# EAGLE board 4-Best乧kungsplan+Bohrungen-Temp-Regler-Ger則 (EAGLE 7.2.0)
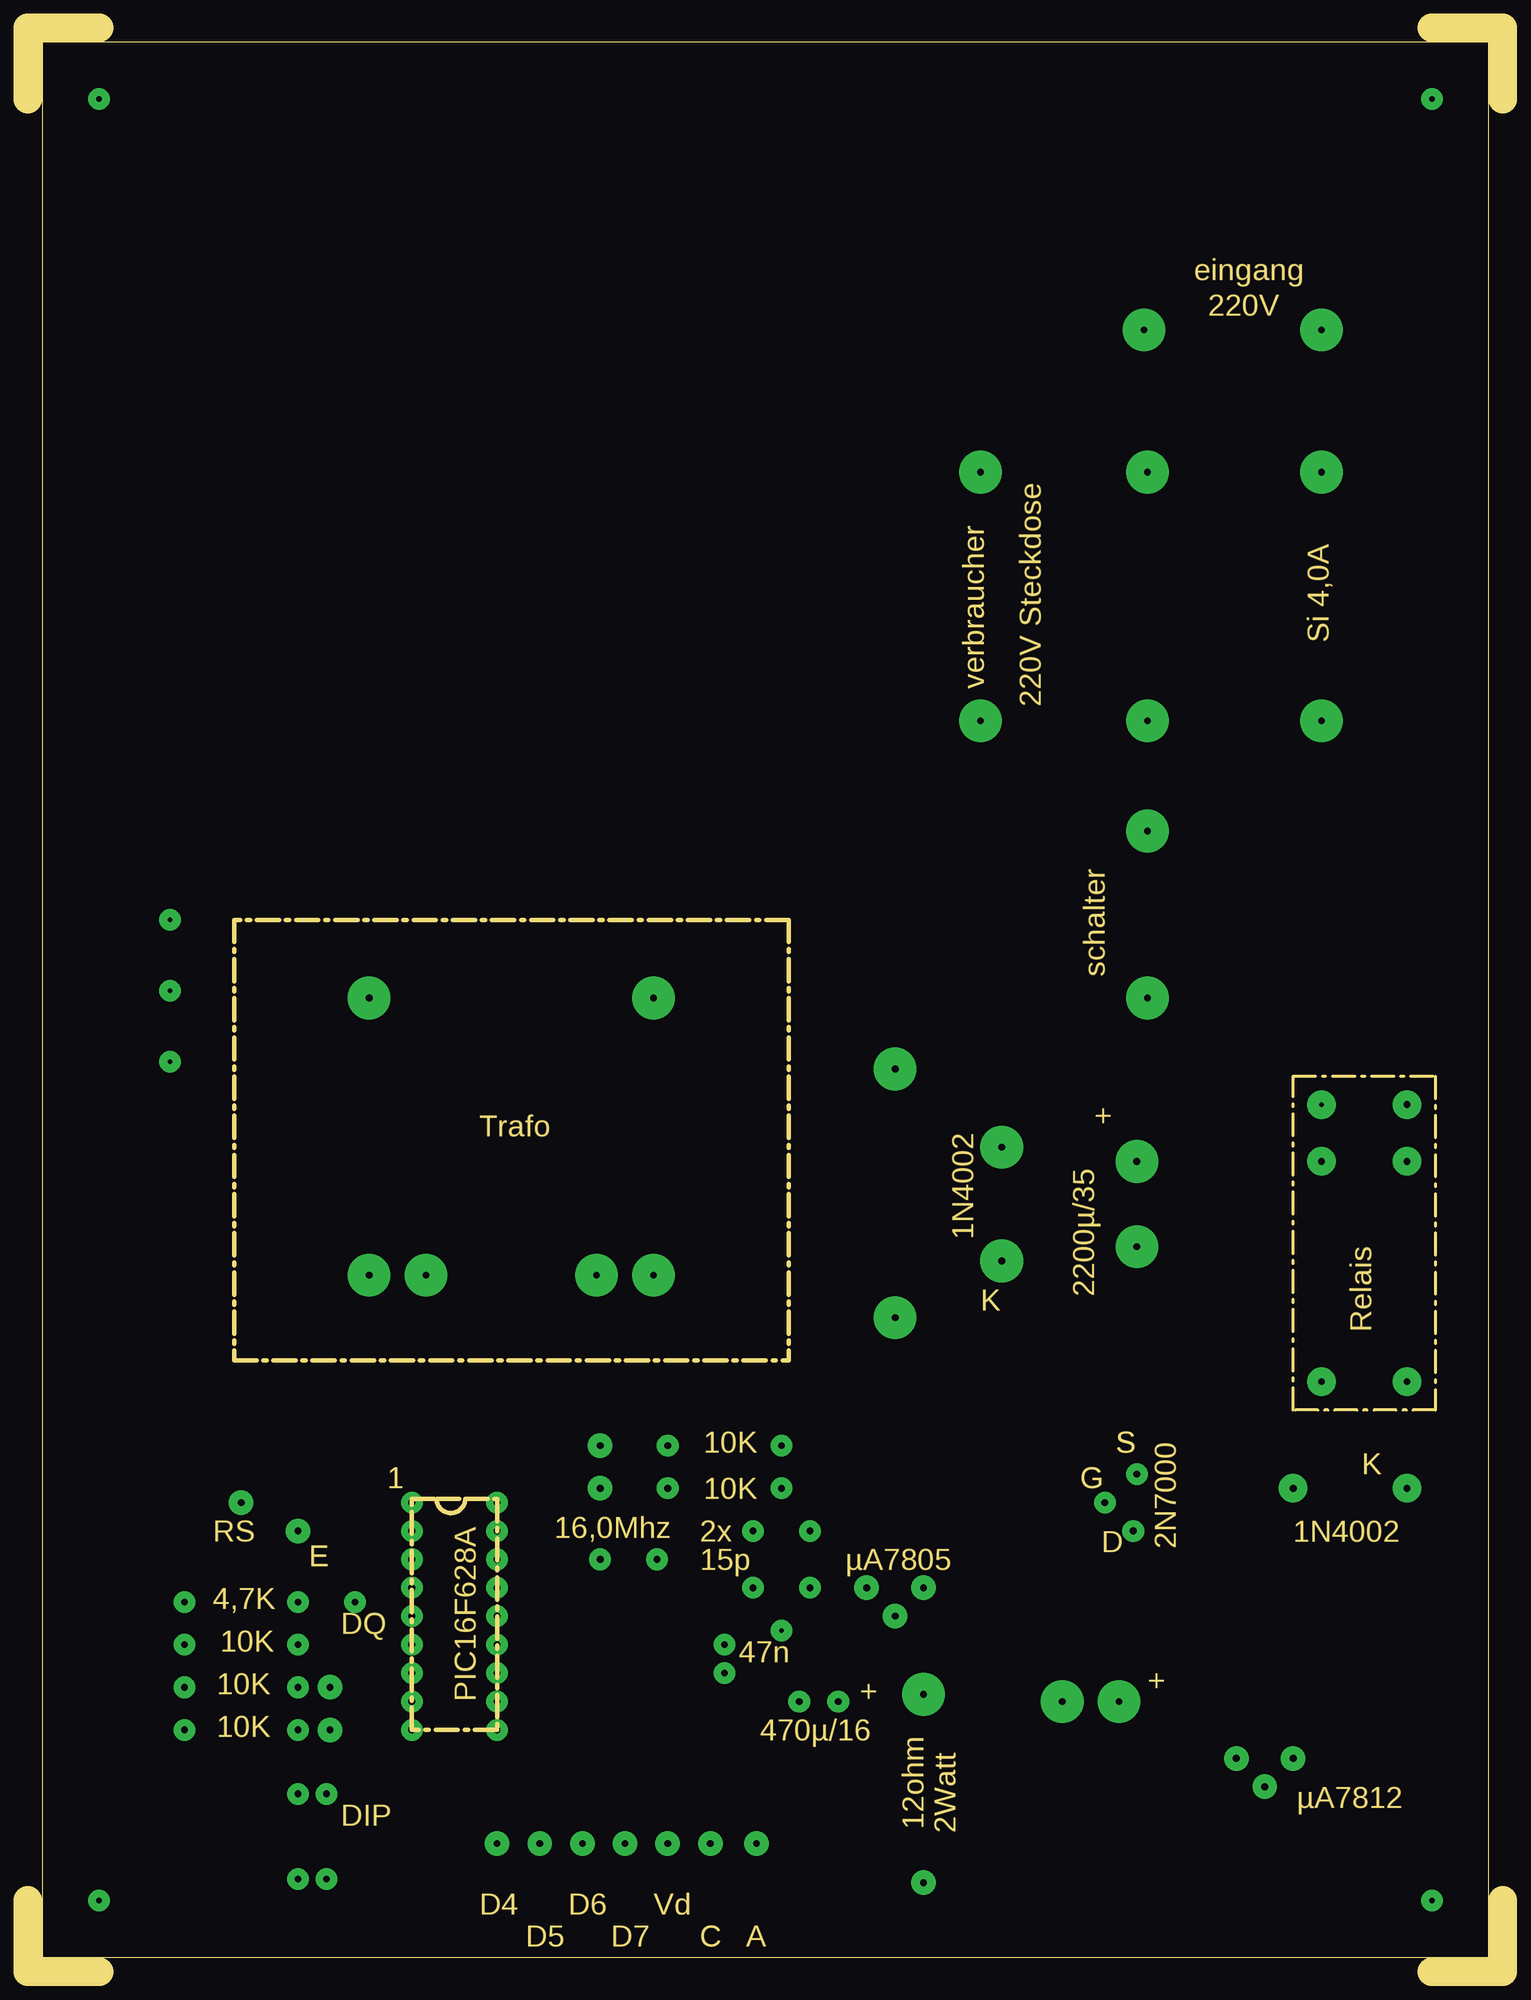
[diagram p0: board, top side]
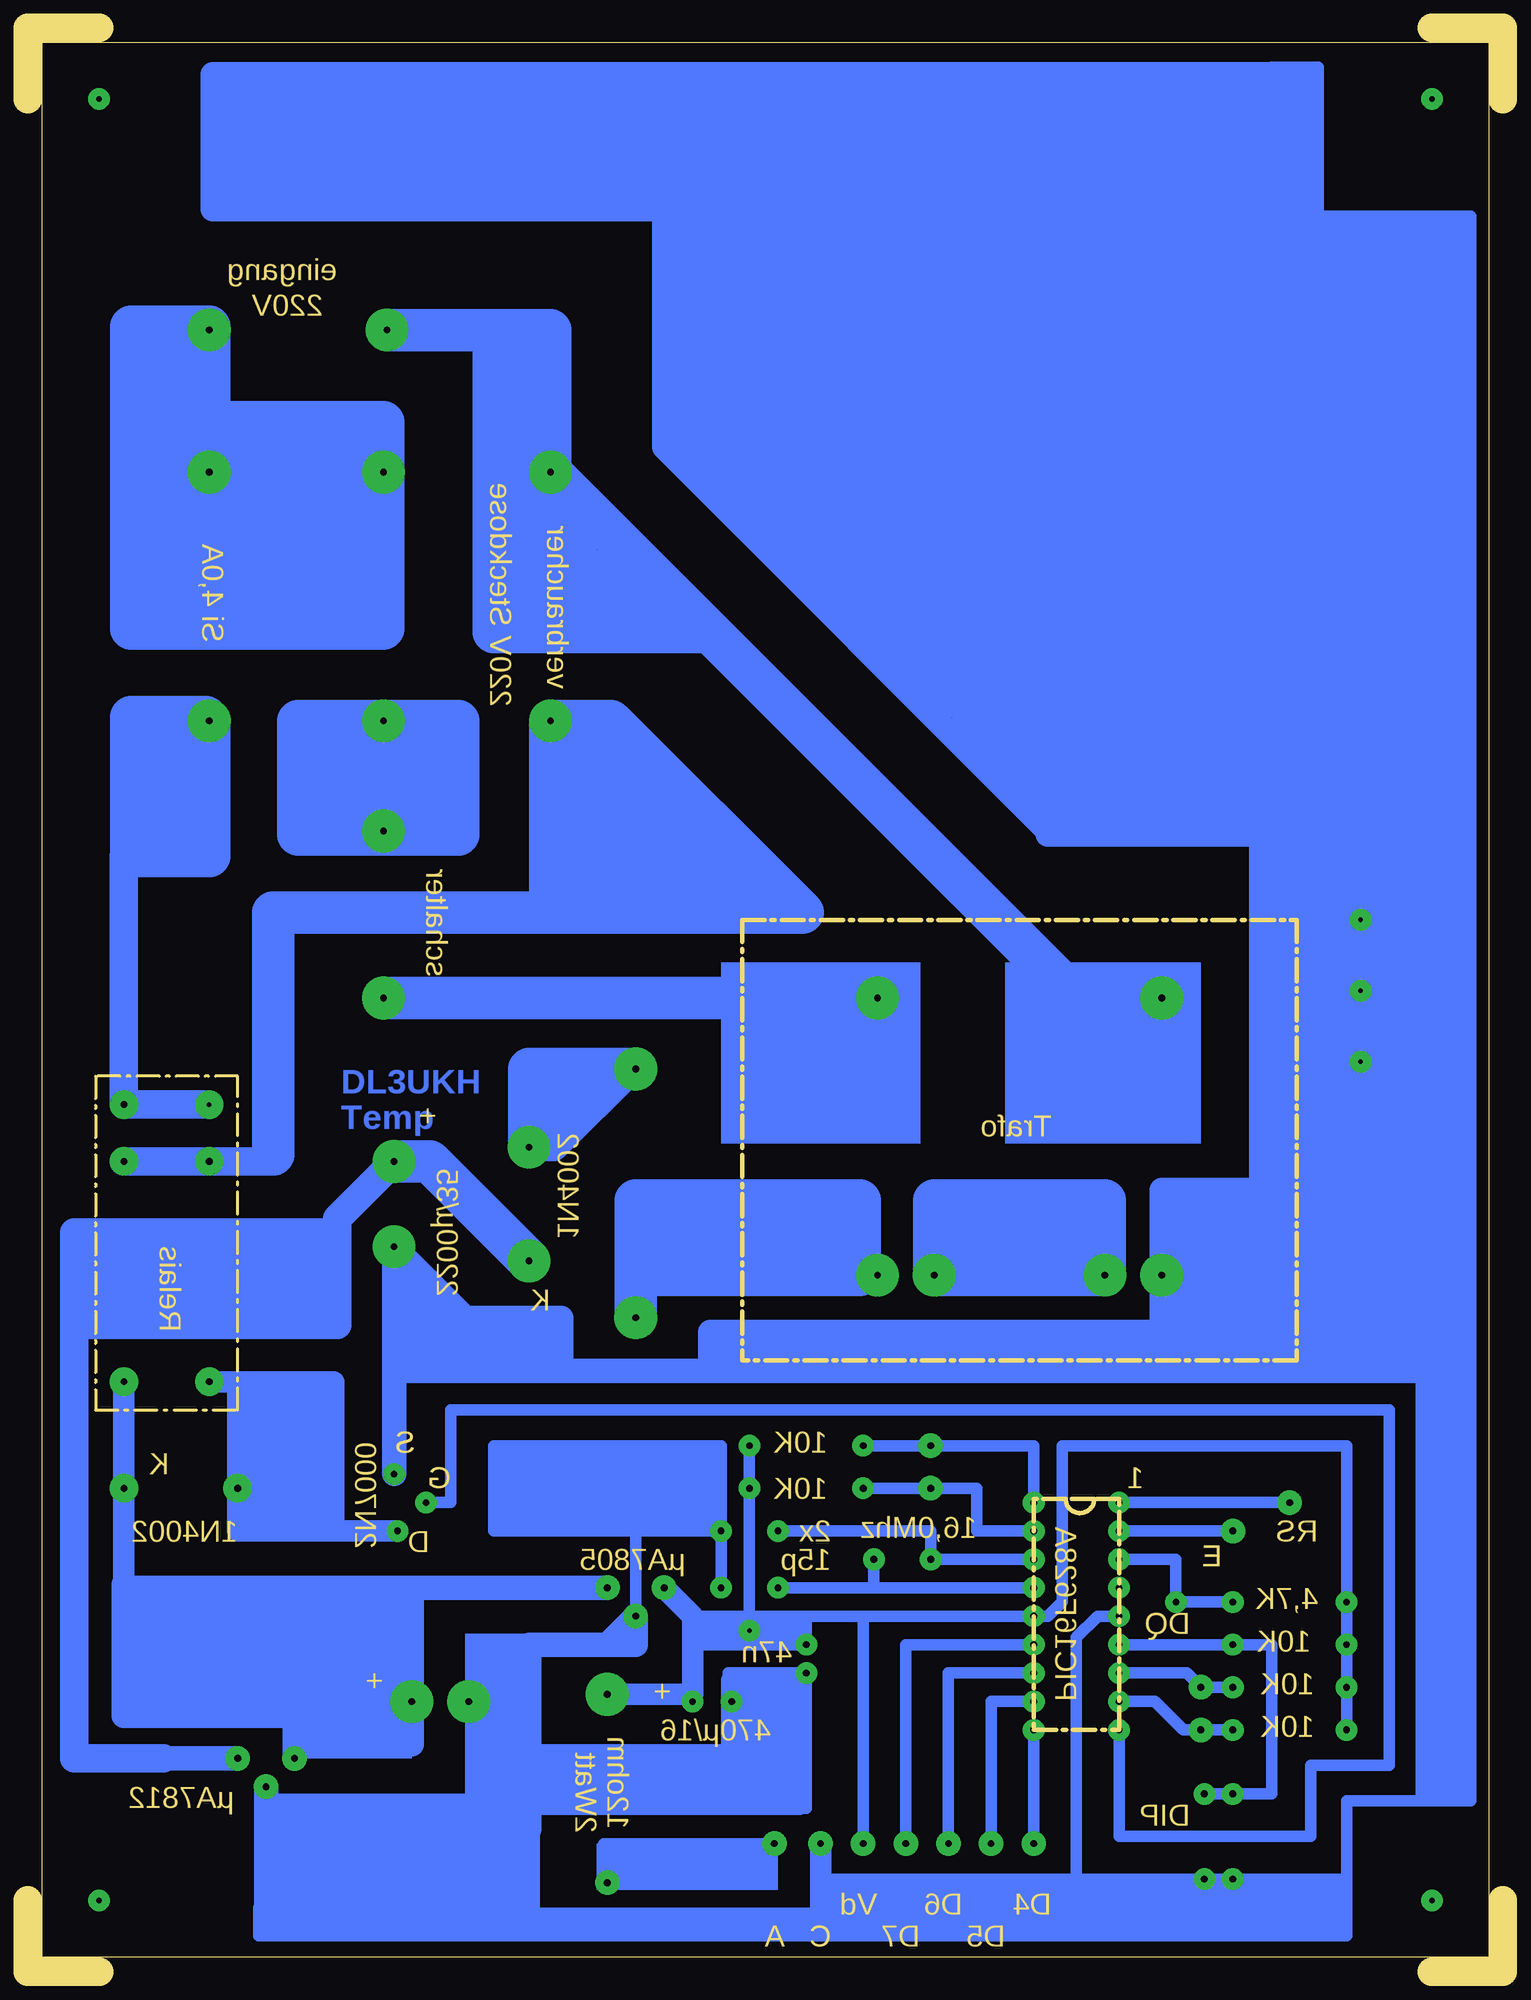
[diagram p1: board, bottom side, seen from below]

Size 131.76 x 173.67 mm. Coordinates in mm from the lower left corner, seen from the top.
Outline: 0,6.35 0,0 6.35,0
Outline: 131.76,6.35 131.76,0 125.41,0
Outline: 0,167.32 0,173.67 6.35,173.67
Outline: 131.76,167.32 131.76,173.67 125.41,173.67
Outline: 36.51,42.23 34.29,42.23 34.29,21.59 41.91,21.59 41.91,42.23 39.05,42.23
Outline: 36.51,42.23 39.05,42.23
Outline: 36.51,42.23 arc180 39.05,42.23
Outline: 1.27,1.27 130.49,1.27 130.49,172.4 1.27,172.4 1.27,1.27
Outline: 67.94,93.98 67.94,54.61 18.41,54.61 18.41,93.98 67.94,93.98
Outline: 113.03,80.01 125.73,80.01 125.73,50.17 113.03,50.17 113.03,80.01
Copper layers (1*16): Top 0.035mm / dielectric 1.5mm / Bottom 0.035mm
Design rules "default": minimum track width 10mil, minimum drill 24mil, track to track 8mil, track to pad 8mil, pad to pad 8mil, via to via 8mil, smd to smd 8mil, copper to edge 40mil, drill to drill 8mil, minimum pad ring 10mil, minimum via ring 8mil, stop-mask expansion 4mil, vias tented up to drill 0mil, thermal gap 10mil

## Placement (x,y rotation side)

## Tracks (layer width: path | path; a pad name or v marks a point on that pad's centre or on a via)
S$1  (via drill 0.5 pad 1.93)
  other vias: 6.35,6.35
S$2  (via drill 0.5 pad 1.93)
  other vias: 6.35,167.32
S$3  (via drill 0.5 pad 1.93)
  other vias: 125.41,167.32
S$4  (via drill 0.5 pad 1.93)
  other vias: 125.41,6.35
S$5  (via drill 0.6 pad 1.93)
  other vias: 72.39,24.13
S$6  (via drill 0.6 pad 3.81)
  Bottom 3.81: v35.56,62.23 v50.8,62.23 50.8,68.9 35.56,68.9 v35.56,62.23
S$7  (via drill 0.6 pad 3.81)
  Bottom 3.81: v100.01,111.76 v100.01,101.92 | v100.01,111.76 100.33,111.76 107.63,111.76 107.63,101.6 93.34,101.6 93.34,111.76 v100.01,111.76
S$8  (via drill 0.6 pad 3.81)
  Bottom 3.81: 77.47,61.91 77.47,62.23 57.47,62.23 57.47,68.9 77.47,68.9 77.47,61.91 | 77.47,61.91 v77.47,58.42
S$9  (via drill 0.6 pad 1.93, 0.6 pad 2.18)
  Bottom 1.016: v41.91,41.91 41.91,46.99 v51.12,46.99 v57.15,46.99
S$10  (via drill 0.6 pad 3.81)
  other vias: 100.01,86.99
S$11  (via drill 0.6 pad 3.81)
  Bottom 3.81: v55.88,86.99 100.01,86.99
S$12  (via drill 0.4 pad 2.54, 0.6 pad 2.54)
  Bottom 2.54: v115.57,77.47 v123.19,77.47 123.19,99.69
S$13  (via drill 0.6 pad 3.81)
  Bottom 3.81: v115.57,111.76 115.57,99.69 122.55,99.69
S$14  (via drill 0.6 pad 2.18)
  Bottom 1.016: v65.09,11.43 80.33,11.43 v80.01,7.94
S$15
  Bottom 3.81: 90.17,146.37 90.17,119.7 71.44,119.7
S$16  (via drill 0.6 pad 1.93)
  Bottom 1.016: v34.29,41.91 19.05,41.91
S$17  (via drill 0.6 pad 1.93, 0.6 pad 2.18)
  Bottom 1.016: v34.29,39.37 v24.13,39.37
S$18  (via drill 0.6 pad 3.81)
  Bottom 3.81: v99.69,146.69 85.09,146.69 v85.09,133.99 38.1,86.99 v30.48,86.99
S$19  (via drill 0.6 pad 3.81)
  other vias: 55.88,62.23
S$20  (via drill 0.6 pad 1.93)
  other vias: 34.29,34.29
S$21  (via drill 0.6 pad 1.93)
  Bottom 1.016: v34.29,31.75 36.2,31.75 38.1,29.84 38.1,12.38
S$22  (via drill 0.6 pad 1.93)
  Bottom 1.016: v34.29,21.59 34.29,12.06 17.14,12.06 17.14,18.41 10.16,18.41 10.16,50.17 93.98,50.17 93.98,41.91 v96.2,41.91
S$23  (via drill 0.6 pad 1.93, 0.6 pad 2.18)
  Bottom 1.016: v24.13,25.4 v26.99,25.4 28.26,26.67 v34.29,26.67
S$24
  Bottom 2.184: 30.8,57.15 70.8,57.15 70.8,54.29
S$25  (via drill 0.6 pad 1.93)
  other vias: 67.31,43.18
S$26  (via drill 0.6 pad 1.93, 0.6 pad 2.18)
  Bottom 1.016: 60.96,5.71 60.96,5.4 | v26.67,8.26 60.96,8.26
  Bottom 1.93: v60.96,11.43 60.96,8.26 60.96,5.71
S$27  (via drill 0.6 pad 1.93, 0.6 pad 2.18)
  Bottom 1.016: v41.91,39.37 46.99,39.37 46.99,43.18 v51.12,43.18 v57.15,43.18
S$28  (via drill 0.6 pad 1.93)
  Bottom 1.016: v41.91,36.83 v51.12,36.83 51.12,39.37 v64.77,39.37
S$29  (via drill 0.6 pad 1.93)
  Bottom 1.016: v41.91,34.29 56.2,34.29 | 56.2,34.29 v56.2,36.83 | 56.2,34.29 v64.77,34.29
S$30  (via drill 0.6 pad 1.93)
  Bottom 1.016: v34.29,29.21 v24.13,29.21 20.64,29.21 20.64,15.88 v26.67,15.88
S$31  (via drill 0.6 pad 1.93, 0.6 pad 2.18)
  Bottom 1.016: v41.91,29.21 53.34,29.21 v53.34,11.43
S$32  (via drill 0.6 pad 1.93, 0.6 pad 2.18)
  Bottom 1.016: v41.91,26.67 49.53,26.67 v49.53,11.43
S$33  (via drill 0.6 pad 1.93, 0.6 pad 2.18)
  Bottom 1.016: v41.91,24.13 45.72,24.13 v45.72,11.43
S$34  (via drill 0.6 pad 1.93, 0.6 pad 2.18)
  Bottom 1.016: v41.91,21.59 v41.91,11.43
S$35  (via drill 0.6 pad 1.93, 0.6 pad 2.18)
  Bottom 1.016: v24.13,21.59 v26.99,21.59 28.57,21.59 31.11,24.13 v34.29,24.13
S$36  (via drill 0.6 pad 3.81)
  Bottom 2.54: 77.79,80.64 84.77,73.66 87.31,73.66
  Bottom 3.81: v77.47,80.64 77.79,80.64 86.99,80.64 v86.99,73.66
S$37  (via drill 0.6 pad 1.93)
  other vias: 24.13,15.88
S$38  (via drill 0.6 pad 3.81)
  Bottom 2.184: v92.39,24.13 87.31,24.13
S$39  (via drill 0.6 pad 3.81)
  Bottom 3.81: 85.09,94.61 109.85,94.61 109.85,73.02 | 85.09,94.61 v85.09,111.76 79.69,111.76 62.55,94.61 85.09,94.61
S$40  (via drill 0.6 pad 2.18, 0.6 pad 3.81)
  Bottom 2.184: v113.03,19.05 119.7,19.05
  Bottom 2.54: 127.63,60.96 104.14,60.96 | 127.63,57.79 127.63,19.05 119.7,19.05 | 127.63,57.79 127.63,59.37 127.63,60.96 | 104.14,60.96 104.14,66.04 | 104.14,66.04 104.14,67.31 v99.06,72.39 | 104.14,60.96 104.14,57.79 127.63,57.79 | 104.14,66.04 127.63,66.04 127.63,60.96
  Bottom 3.81: v99.06,72.39 95.88,72.39 v86.99,63.5
S$41  (via drill 0.6 pad 1.93, 0.6 pad 2.18)
  Bottom 1.016: 21.59,53.34 7.3,53.34 | 7.3,53.34 7.3,15.24 | 7.3,15.24 13.97,15.24 13.97,8.26 | 62.23,24.13 v62.23,26.67 69.21,26.67 69.21,24.13 | 62.23,24.13 v68.9,24.13 | v69.85,39.37 v69.85,34.29 | 77.47,39.37 v69.85,39.37 | v77.47,31.75 77.47,39.37 | 86.99,5.08 86.99,13.02 | 38.1,5.08 86.99,5.08 | 38.1,5.08 38.1,12.06 | 86.99,5.08 111.12,5.08 | 62.23,24.13 62.23,14.61 69.21,14.61 | 26.67,5.08 24.13,5.08 | 24.13,5.08 13.97,5.08 | v24.13,8.26 26.67,8.26 26.67,5.08 | 38.1,5.08 26.67,5.08 | 13.97,8.26 13.97,5.08 | v24.13,8.26 24.13,5.08 | v69.85,39.37 69.85,46.99 90.17,46.99 90.17,39.37 77.47,39.37 | v24.13,8.26 13.97,8.26 | 7.3,15.24 2.86,15.24 2.86,53.34 | 2.86,53.34 7.3,53.34 | 2.86,53.34 2.86,156.84 16.51,156.84 16.51,170.18 20.64,170.18 | 13.97,5.08 13.97,3.17 111.12,3.17 111.12,5.71
  Bottom 1.93: 68.9,19.37 v68.9,24.13 68.9,26.04 | 68.9,19.37 86.68,19.37 | 68.9,19.37 68.9,14.92 | 86.99,29.21 86.99,24.13 | 68.9,14.92 86.99,14.92 | 68.9,14.92 62.87,14.92
  Bottom 2.184: 110.49,12.7 v110.49,16.51 | 80.01,29.21 v77.47,31.75 77.47,29.21 80.01,29.21 | 80.01,29.21 86.99,29.21 86.99,14.92 86.99,13.02 86.99,12.7 110.49,12.7 | 110.49,12.7 110.49,5.71
S$42  (via drill 0.6 pad 2.18, 0.6 pad 2.54, 0.6 pad 3.81)
  Bottom 1.016: v80.01,34.29 82.55,34.29
  Bottom 1.93: v123.19,52.71 123.19,34.61 123.19,29.21 115.57,29.21
  Bottom 2.184: 115.57,22.86 115.57,29.21 | v97.47,24.13 97.47,34.29 | 107.95,22.86 v107.95,19.05 | 107.95,22.86 115.57,22.86 | 107.95,22.86 97.47,22.86 v97.47,24.13 | v97.47,24.13 97.47,20.32 | 97.47,34.29 v80.01,34.29 | 97.47,34.29 123.19,34.29 | 123.19,34.29 123.19,34.61 | 115.57,22.86 123.19,22.86 123.19,34.29
S$43  (via drill 0.6 pad 1.93, 0.6 pad 2.54)
  Bottom 1.93: 104.46,39.37 104.46,52.71 113.03,52.71 | 104.46,39.37 103.82,39.37 v98.74,39.37 | 113.03,52.71 v115.57,52.71 | 113.03,52.71 v113.03,43.18 113.03,39.37 104.46,39.37
S$44  (via drill 0.6 pad 2.54)
  Bottom 2.54: v123.19,72.39 v115.57,72.39 109.85,72.39
S$45
  Bottom 3.81: 115.89,112.08 122.55,112.08 122.55,100.01
S$46  (via drill 0.6 pad 1.93, 0.6 pad 2.18)
  Bottom 1.016: v13.97,21.59 v13.97,33.02 13.97,46.99 39.37,46.99 39.37,33.02 40.64,31.75 v41.91,31.75 57.15,31.75 | 57.15,31.75 62.23,31.75 | 62.23,31.75 67.31,31.75 | 67.31,31.75 72.07,31.75 | 62.23,31.75 v62.23,29.21 72.07,29.21 | 57.15,31.75 v57.15,11.43 | v67.31,46.99 67.31,31.75
S$47  (via drill 0.6 pad 2.54)
  other vias: 123.19,43.18
S$48  (via drill 0.6 pad 3.81)
  Bottom 3.81: 115.57,147 122.55,147 122.55,133.99 | v115.57,146.69 v115.57,133.99 | v115.57,133.99 v100.01,133.99 | v115.57,133.99 122.55,133.99 | 122.55,133.99 122.55,120.02 100.01,120.02 100.01,138.43 114.3,138.43
S$49  (via drill 0.4 pad 1.93)
  other vias: 12.7,93.98
S$50  (via drill 0.4 pad 1.93)
  other vias: 12.7,87.63
S$51  (via drill 0.4 pad 1.93)
  other vias: 12.7,81.28
S$52  (via drill 0.6 pad 2.18, 0.6 pad 3.81)
  Bottom 1.93: v74.93,34.29 72.39,31.75 72.39,24.77 v80.01,24.77
S$53  (via drill 0.4 pad 1.93)
  other vias: 67.31,30.48
S$56  (via drill 0.6 pad 2.18)
  other vias: 19.05,41.91
S$58  (via drill 0.6 pad 1.93)
  other vias: 13.97,29.21
S$59  (via drill 0.6 pad 1.93, 0.6 pad 3.81)
  Bottom 1.016: v30.48,62.23 30.48,62.55
  Bottom 2.184: 99.06,53.66 v99.06,64.77 92.71,58.42 84.14,58.42 84.14,53.66 | 30.48,53.98 v30.48,62.23 | 30.48,53.66 84.14,53.66 | 84.14,53.66 99.06,53.66 | 99.06,53.66 v99.06,44.45 | v30.48,62.23 21.59,62.23 | 21.59,69.85 21.59,62.23 | v30.48,62.23 30.48,69.85 21.59,69.85 | 21.59,62.23 21.59,53.98 30.48,53.98 | 30.48,53.66 30.48,53.98 | 7.94,53.66 30.48,53.66 | 21.59,69.85 21.59,101.6 | 3.81,120.02 21.59,120.02 21.59,101.6 | 21.59,101.6 40.64,101.6 40.64,101.92 74.93,136.21 74.93,157.48 115.25,157.48 115.25,169.55 19.05,169.55
S$60  (via drill 0.6 pad 1.93)
  other vias: 13.97,25.4
S$63  (via drill 0.6 pad 1.93)
  Bottom 1.016: v24.13,33.02 v29.21,33.02 29.21,36.83 v34.29,36.83
(copper drawn outside any net)
  shapes: Bottom area x70

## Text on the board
Bottom: DL3UKH | Temp
Pads: AUF BESTÜCKUNGS-SEITE GESEHEN
Dimension: eingang | 220V | Trafo 1,0mm | µA7812 + µA7805 1,0mm | Si 4,0A | verbraucher | 220V Steckdose | schalter | K | + | Trafo | 1N4002 | 2200µ/35 | K | Relais | und µA7812 | 10K | S | S | K | 1 | G | 10K | 1N4002 | RS | 16,0Mhz | 2x | 2N7000 | D | E | 15p | µA7805 | 4,7K | DQ | 10K | 47n | + | 10K | PIC16F628A | + | 10K | 470µ/16 | µA7812 | DIP | 12ohm | 2Watt | D4 | D6 | Vd | D5 | D7 | C | A
tOrigins: Alles mit 0,8mm vorbohren ! | 2N7000 | Aufbohren: | Diode 1N4002 1,0mm | Sicherungshalter 1,5mm | 4Stck. Befestigungsbohr... 3,2mm | 12ohm/2Watt 1,0mm | Relais 1,0mm | S | D | Elkos 1,0mm | G | Si 315mA | 1N4002 | Leiterplatte: | 1,5mm dick | Cevausit | Katode | Anode | IC's | 1 | Die Aussparung | Links oben ist | muß mit dem | immer PIN 1 | Bauelement | und dem Bestück- | Si 315mA | ungsplan | überein stimmen. | µA7805 | Eing. | Eing. | Ausg. | Eing. | 1000µ/35V | Masse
